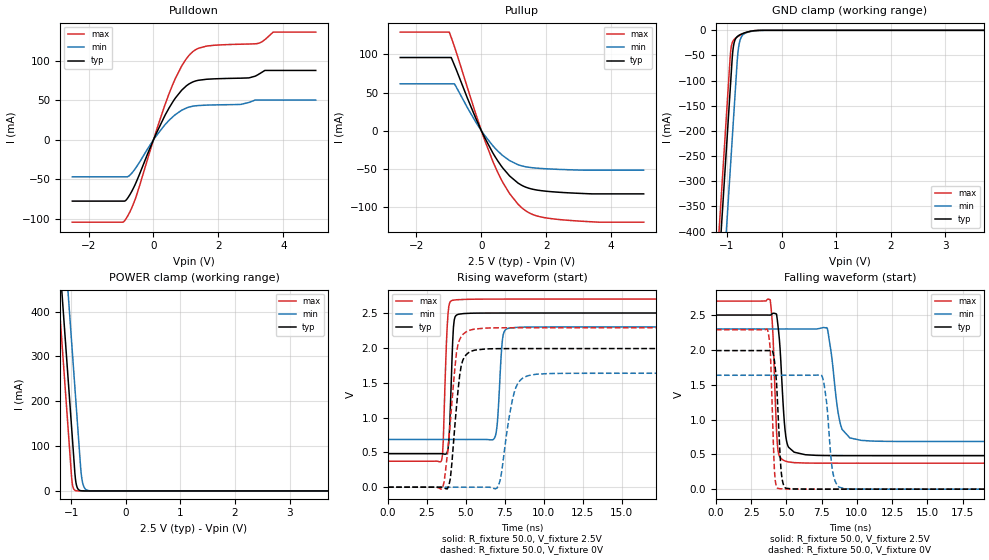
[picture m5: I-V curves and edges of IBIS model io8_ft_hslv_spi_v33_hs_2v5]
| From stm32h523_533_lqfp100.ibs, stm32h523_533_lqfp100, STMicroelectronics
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[Model]   io8_ft_hslv_spi_v33_hs_2v5
Model_type I/O
Polarity   Non-Inverting
Enable   Active-Low
| CAP_THRESHOLD on pad IOFT is "UDTCAPC" :
| Rising=20.0% of vddiom   Falling=80.0% of vddiom
| C_comp min and max val. don't necessarily correlate with the min and max pvt
| but are the smallest and greatest pad capacitance found.
| var   typ   min   max
C_comp   3.86841pF  3.83555pF  3.96274pF
|C_comp_pullup   2.45375pF  2.33560pF  2.34205pF
|C_comp_pulldown   1.41466pF  1.49995pF  1.62069pF
Vinl = 690.0mV
Vinh = 1.89V
Vmeas = 1.25V   | Reference voltage for timing measurements
Cref  = 50.0pF   | Timing specification test load capacitance value
Rref  = 100.0MOhm   | Timing specification test load resistance value
Vref  = 1.25V   | Timing specification test load voltage
[Model Spec]
| TIME_THRESHOLD on pin ZIV33M is "CMOS" :
| Rising=40.0% of vddiom   Falling=60.0% of vddiom
Vinl 978.80000mV 906.80000mV 1.05480V
Vinh 1.39920V 1.29220V 1.48720V
| variable   typ   min   max
[Temperature Range] 25.0 125.0 -40.0
| variable   typ   min   max
[Voltage Range] 2.5V 2.3V 2.7V
| variable   typ   min   max
[POWER Clamp Reference] 2.5V 2.3V 2.7V
| variable   typ   min   max
[GND Clamp Reference] 0V 0V 0V
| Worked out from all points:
|   slope of the pulldown table from 0 to 0.375 V, typ, clamps not added: 11.5 ohm
|   slope of the pullup table from 0 to 0.375 V, typ, clamps not added: 12.3 ohm
|   GND clamp passes 1 mA (typ) near -0.52 V on its own axis
|   POWER clamp passes 1 mA (typ) near -0.84 V on its own axis
|   rising waveform, R_fixture 50.0, V_fixture 2.5V: 20-80 % time 193ps typ, 242ps min, 213ps max; typ from 0.481 V to 2.5 V
|   falling waveform, R_fixture 50.0, V_fixture 2.5V: 20-80 % time 366ps typ, 588ps min, 259ps max; typ from 2.5 V to 0.481 V
|   rising waveform, R_fixture 50.0, V_fixture 0V: 20-80 % time 476ps typ, 686ps min, 546ps max; typ from 0 V to 1.99 V
|   falling waveform, R_fixture 50.0, V_fixture 0V: 20-80 % time 303ps typ, 420ps min, 224ps max; typ from 1.99 V to 0 V
[POWER Clamp]
-2.5V     2.708A     2.899A     2.597A
-1.23V    548.8mA    740.2mA    437.5mA
-1.16V    429.8mA    621.2mA    318.5mA
-1.12V    361.8mA    553.2mA    250.5mA
-1.03V    208.8mA    400.2mA    97.53mA
-980mV    123.8mA    315.2mA    17.95mA
-920mV    26.3mA     213.2mA    906uA
-880mV    5.543mA    145.2mA    123.7uA
-810mV    363.5uA    33.6mA     3.797uA
-770mV    76.62uA    10.47mA    518.8nA
-700mV    5.026uA    1.361mA    16.09nA
5V        0A         0A         0A
[GND Clamp]
-2.5V     -2.77A     -2.931A    -2.704A
-1.21V    -576.8mA   -738.1mA   -511.3mA
-950mV    -134.8mA   -296.1mA   -69.34mA
-920mV    -83.82mA   -245.1mA   -32.48mA
-900mV    -50.56mA   -211.1mA   -24.02mA
-880mV    -31.31mA   -177.1mA   -19.85mA
-850mV    -18.7mA    -126.1mA   -16.34mA
-800mV    -11.46mA   -46.18mA   -12.45mA
-750mV    -8.203mA   -16.63mA   -9.325mA
-650mV    -4.063mA   -4.987mA   -4.427mA
-360mV    -35.05uA   -165.1uA   -9.564uA
5V        7.96nA     1.282uA    294pA
| variable   typ   min   max
[Pullup Reference] 2.5V 2.3V 2.7V
| variable   typ   min   max
[Pulldown Reference] 0V 0V 0V
[Pullup]
-2.5V     95.83mA    61.44mA    129.1mA
-990mV    95.83mA    61.44mA    129.1mA
-930mV    95.83mA    61.44mA    122.2mA
-830mV    85.75mA    61.44mA    110.1mA
-170mV    16.04mA    11.14mA    21.66mA
350mV     -28.77mA   -19.46mA   -39.69mA
610mV     -45.89mA   -30.7mA    -63.55mA
870mV     -59.15mA   -39.06mA   -82.32mA
1.28V     -72.18mA   -46.35mA   -102mA
1.66V     -77.19mA   -48.75mA   -110.8mA
2.28V     -80.15mA   -50.35mA   -115.7mA
5V        -82.59mA   -51.55mA   -119.6mA
[Pulldown]
-2.5V     -77.63mA   -46.85mA   -104.3mA
-870mV    -77.24mA   -46.85mA   -101.4mA
-550mV    -55.3mA    -35.88mA   -73.72mA
90mV      8.401mA    5.299mA    11.79mA
610mV     49.03mA    29.76mA    71.69mA
870mV     62.92mA    37.48mA    93.62mA
1.23V     73.63mA    42.72mA    112.2mA
1.64V     76.78mA    44.01mA    118.8mA
2.7V      78.15mA    44.99mA    121.2mA
3.22V     82.58mA    50.35mA    122.2mA
3.69V     87.93mA    50.35mA    136.5mA
5V        87.93mA    50.35mA    136.5mA
[Ramp]
dV/dt_r 1.19372V/474.20362ps 981.18245mV/681.1978ps 1.37325V/541.98861ps
dV/dt_f 1.21165V/362.81832ps 969.2616mV/587.26495ps 1.39628V/256.96908ps
R_load = 50.0
| Removed startup time: 0s 0s 0s  .
| Removed end time: 23.75ns.
[Rising Waveform]
R_fixture   = 50.0
V_fixture   = 2.5V
V_fixture_min = 2.3V
V_fixture_max = 2.7V
0s        480.6mV    684.6mV    372.9mV
3.45ns    481mV      684.6mV    394.3mV
3.9ns     642.3mV    684.6mV    2.593V
4.1ns     1.792V     684.6mV    2.679V
4.35ns    2.461V     684.6mV    2.689V
6.85ns    2.5V       710.2mV    2.7V
7.05ns    2.5V       1.01V      2.7V
7.35ns    2.5V       2.124V     2.7V
7.65ns    2.5V       2.274V     2.7V
23.75ns   2.5V       2.3V       2.7V
| Removed startup time: 0s 0s 0s  .
| Removed end time: 38.75ns.
[Falling Waveform]
R_fixture   = 50.0
V_fixture   = 2.5V
V_fixture_min = 2.3V
V_fixture_max = 2.7V
0s        2.5V       2.3V       2.7V
3.85ns    2.499V     2.3V       2.719V
4.05ns    2.525V     2.3V       2.187V
4.35ns    2.433V     2.3V       655.1mV
4.85ns    961.9mV    2.3V       408.9mV
5ns       699.3mV    2.3V       397.9mV
7.9ns     482.3mV    2.308V     373.2mV
8.75ns    481.3mV    1.006V     373mV
9.5ns     480.9mV    736.2mV    373mV
38.75ns   480.6mV    684.6mV    372.9mV
| Removed startup time: 0s 0s 0s  .
| Removed end time: 38.6ns.
[Rising Waveform]
R_fixture   = 50.0
V_fixture   = 0V
V_fixture_min = 0V
V_fixture_max = 0V
0s        189.1nV    426nV      147.2nV
3.5ns     -1.255mV   -120.5nV   -10.76mV
4ns       122.4mV    -293.1nV   948.1mV
4.4ns     1.168V     -301nV     1.941V
4.7ns     1.746V     -263.2nV   2.162V
5.4ns     1.956V     -2.918uV   2.262V
7.1ns     1.988V     29.41mV    2.287V
8.1ns     1.989V     1.357V     2.288V
9.1ns     1.989V     1.606V     2.289V
38.6ns    1.99V      1.635V     2.289V
| Removed startup time: 0s 0s 0s  .
| Removed end time: 23.75ns.
[Falling Waveform]
R_fixture   = 50.0
V_fixture   = 0V
V_fixture_min = 0V
V_fixture_max = 0V
0s        1.99V      1.635V     2.289V
3.65ns    1.99V      1.635V     2.291V
3.85ns    1.993V     1.635V     2.01V
4.15ns    1.839V     1.635V     258.4mV
4.4ns     1.106V     1.635V     11.01mV
4.85ns    36.04mV    1.635V     3.221mV
7.5ns     376.5uV    1.632V     194.2uV
8.25ns    229.4uV    291.8mV    123.6uV
8.75ns    176.4uV    26.46mV    96.17uV
23.75ns   2.26uV     19.2uV     458.1nV
